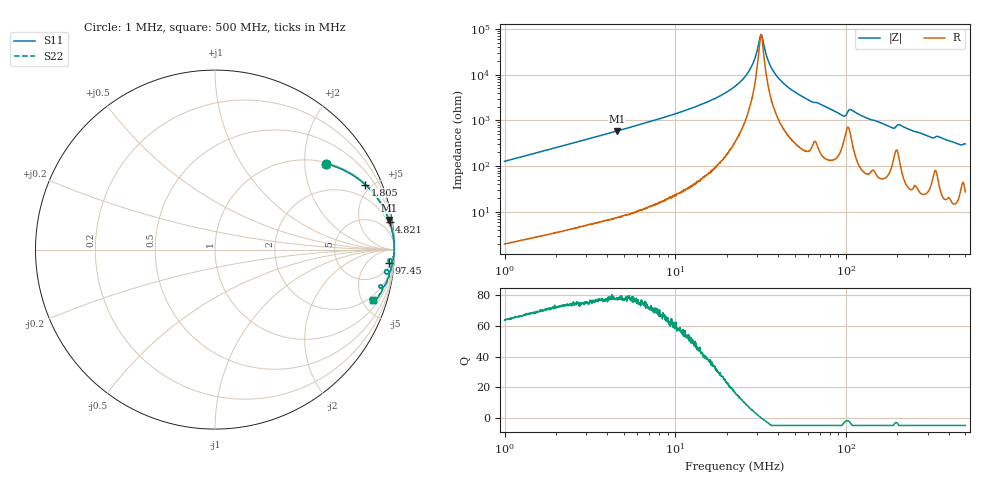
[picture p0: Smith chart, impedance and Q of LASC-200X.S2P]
!s-Parameter Generated by FASTRON Sdn. Bhd.
!FASTRON P/N : LASC-200X
!Keysight Technologies,E4991B,MY54100416,A.01.15
!Date: Tue Mar 17 13:51:39 2026
!Version  : Rev00 Tue Mar 17 13:51:39 2026
!Data & Calibration Information:
!PortZ  Port1:50+j0  Port2:50+j0
!When reading, reference impedance value at option line is always used.
! Remarks : This data is being provided solely for informational purposes.
!Freq	S11	S21	S12	S22
# Hz S dB R 50
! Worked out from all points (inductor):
!   1601 points, 1 MHz to 500 MHz, reference 50 ohm
!   read as one part in series: L = 20.3 uH near 1.032 MHz
!   highest Q = 78.5 at 4.549 MHz (marker M1), where L = 20.5 uH
!   self-resonance near 31.72 MHz
!   S11 on the Smith chart (normalised r, x): 1 MHz: 1.04, +2.55; 1.805 MHz: 1.07, +4.60; 4.821 MHz: 1, +12; 97.45 MHz: 9, -24; 500 MHz: 1.55, -6.08
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1000000  -2.14 37.7  -4.27 -51.4  -4.27 -51.4  -2.14 37.7
1804688  -0.80 23.4  -8.02 -65.8  -8.02 -65.8  -0.80 23.4
2820919  -0.35 15.5  -11.47 -73.7  -11.47 -73.7  -0.35 15.5
4548560  -0.14 9.7  -15.50 -79.6  -15.50 -79.6  -0.14 9.7
4821440  -0.13 9.1  -16.01 -80.2  -16.01 -80.2  -0.13 9.1
7957584  -0.05 5.3  -20.62 -83.8  -20.62 -83.8  -0.05 5.3
1.534122e7  -0.02 2.3  -28.01 -86.2  -28.01 -86.2  -0.02 2.3
2.236068e7  -0.01 1.0  -34.90 -85.6  -34.90 -85.6  -0.01 1.0
2.757879e7  -0.01 0.4  -42.74 -80.0  -42.74 -80.0  -0.01 0.4
2.934708e7  -0.01 0.2  -47.40 -72.6  -47.40 -72.6  -0.01 0.2
3.122875e7  -0.01 0.1  -55.80 -37.3  -55.80 -37.3  -0.01 0.1
3.184116e7  -0.01 -0.0  -57.49 0.8  -57.49 0.8  -0.01 -0.0
3.549939e7  -0.01 -0.3  -44.98 75.6  -44.98 75.6  -0.01 -0.3
3.957791e7  -0.01 -0.6  -39.09 81.9  -39.09 81.9  -0.01 -0.6
4.750454e7  -0.02 -1.2  -33.60 84.0  -33.60 84.0  -0.02 -1.2
6.307767e7  -0.04 -2.2  -28.14 81.9  -28.14 81.9  -0.04 -2.2
9.745486e7  -0.24 -4.3  -22.07 67.9  -22.07 67.9  -0.24 -4.3
1.069764e8  -0.14 -3.2  -24.80 72.5  -24.80 72.5  -0.14 -3.2
1.77937e8  -0.18 -7.5  -17.60 77.3  -17.60 77.3  -0.18 -7.5
2.054376e8  -0.24 -6.9  -18.32 73.6  -18.32 73.6  -0.24 -6.9
3.125075e8  -0.38 -12.8  -13.08 72.5  -13.08 72.5  -0.38 -12.8
5e8  -0.67 -17.6  -10.36 67.3  -10.36 67.3  -0.67 -17.6
